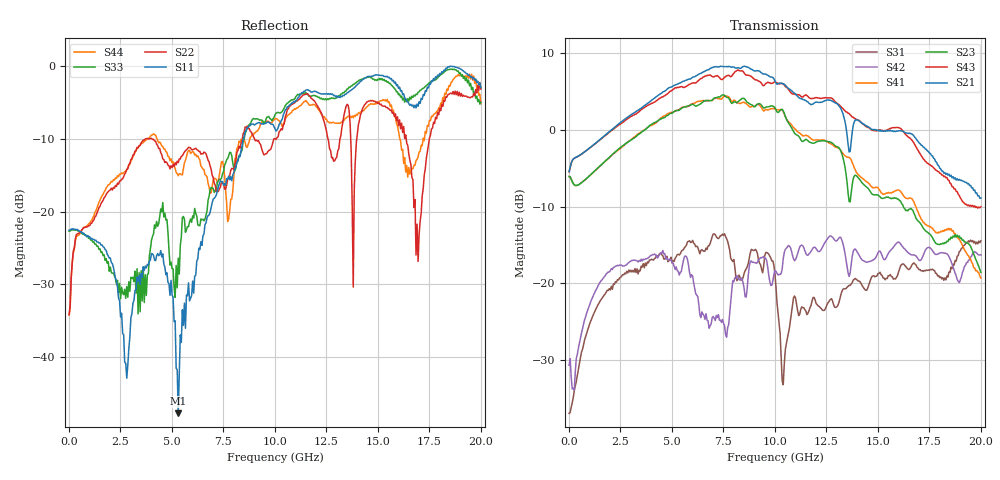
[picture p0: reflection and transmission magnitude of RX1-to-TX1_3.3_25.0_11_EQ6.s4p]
!Agilent Technologies,N5225A,MY51451112,A.09.50.13
!Agilent N5225A: A.09.50.13
!Date: Wednesday, January 31, 2018 11:03:59
!Correction: S11(Full 4 Port(1,2,3,4))
!S12(Full 4 Port(1,2,3,4))
!S13(Full 4 Port(1,2,3,4))
!S14(Full 4 Port(1,2,3,4))
!S21(Full 4 Port(1,2,3,4))
!S22(Full 4 Port(1,2,3,4))
!S23(Full 4 Port(1,2,3,4))
!S24(Full 4 Port(1,2,3,4))
!S31(Full 4 Port(1,2,3,4))
!S32(Full 4 Port(1,2,3,4))
!S33(Full 4 Port(1,2,3,4))
!S34(Full 4 Port(1,2,3,4))
!S41(Full 4 Port(1,2,3,4))
!S42(Full 4 Port(1,2,3,4))
!S43(Full 4 Port(1,2,3,4))
!S44(Full 4 Port(1,2,3,4))
!S4P File: Measurements: <S11,S12,S13,S14>,
!<S21,S22,S23,S24>,
!<S31,S32,S33,S34>,
!<S41,S42,S43,S44>:
# Hz S  RI  R 50
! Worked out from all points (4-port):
!   401 points, 10 MHz to 20 GHz, reference 50 ohm
!   strongest paths, dB at 10 MHz, 5.008 GHz, 10.01 GHz, 15 GHz, 20 GHz:
!     S21: -5.4, 5.6, 6.4, 0.0, -8.9
!     S43: -5.5, 5.2, 6.3, 0.0, -10.0
!     S23: -6.1, 2.2, 2.9, -8.5, -18.5
!     S41: -6.1, 2.3, 2.7, -7.5, -19.3
!     S42: -30.7, -17.3, -18.3, -16.0, -16.3
!     S31: -36.9, -17.4, -18.9, -18.7, -14.4
!   lowest |S11| = -47.8 dB at 5.307 GHz (marker M1), VSWR 1.01, Z = 49.6 - j0.00292 ohm
!   |S11| at or under -10 dB: start of sweep to 8.468 GHz
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1e7  -0.0743 -0.00317  -7.86e-05 0.00066  0.0137 0.000863  -3.13e-05 0.00042
     0.5358 0.0098  -0.0132 0.0144  -0.4976 0.00155  0.0262 0.0117
     0.0142 0.000662  -0.000151 0.000237  -0.0733 -0.00411  4.59e-05 0.000248
     -0.4976 0.0023  0.0265 0.0124  0.5338 0.00858  -0.013 0.0143
5.30735e9  -0.00408 -2.95e-05  0.0285 -0.00431  0.096 0.1374  0.0295 -0.014
           -0.8554 -1.808  0.125 -0.1784  0.7969 1.078  0.1224 0.00784
           0.09 0.1261  0.0329 -0.00103  0.0385 0.0283  0.0404 -0.0103
           1.08 0.8147  0.1188 0.0144  -1.418 -1.249  0.0639 -0.1649
7.10645e9  -0.0217 0.1243  0.016 -0.0174  0.1321 0.0816  0.00472 -0.0328
           -2.581 0.1361  0.1193 -0.0935  1.578 -0.3789  0.0457 0.0243
           0.1709 0.1188  0.0251 -0.0228  0.0142 0.1393  0.0153 -0.0451
           1.285 -0.9773  0.0572 -0.00365  -1.918 1.176  0.1038 -0.1333
8.8056e9  0.0187 0.3913  0.0121 -0.0144  0.1137 0.0909  -0.00615 -0.0153
          -0.6324 2.425  -0.0884 0.3457  0.139 -1.466  0.0336 0.1281
          0.1272 0.094  0.00135 -0.0235  0.0629 0.3957  -0.0141 -0.0256
          -0.511 -1.314  -0.00323 0.1391  0.6625 2.15  0.2532 0.2037
1.270365e10  0.2728 0.5894  -0.0373 -0.0098  0.0219 0.069  -0.0311 0.00769
             1.35 -0.7851  0.1598 0.2096  -0.6158 0.5617  0.1829 0.1036
             0.0239 0.0752  -0.0308 -0.0104  0.3937 0.4514  -0.0426 -0.00188
             -0.1363 0.8038  0.1784 0.0998  0.3745 -1.575  0.2467 -0.3292
1.665168e10  0.5166 0.1354  -0.0276 0.0163  -0.0525 0.1083  -0.00318 0.0373
             -0.8672 -0.3675  0.00945 0.1718  0.2676 0.1427  0.0924 0.1124
             -0.0563 0.1194  -0.0261 0.00427  0.5994 -0.1772  -0.00827 0.0369
             0.3135 -0.1701  0.1064 0.1105  -0.5432 0.6658  -0.1123 -0.1623
2e10  0.7116 0.0649  0.023 0.0349  -0.0787 0.1648  0.0347 0.0209
      -0.03 0.3596  0.6936 0.0755  0.0586 -0.1028  0.153 0.042
      -0.0801 0.172  0.00637 0.0478  0.5651 -0.0284  0.0477 0.0206
      -0.0754 -0.078  0.1466 0.0459  0.2834 0.1398  -0.1525 -0.5327
